FUNCTION_BLOCK FB62
TITLE =Set Position Must
//*****************************************************************************
//* maxon motor ag
//* R&D
//* all rights reserved
//*****************************************************************************
//* Summary:  Write demand value of position
//*
//* Remarks:
//*
//* Created under: STEP7 REV5.2+SP1
//*****************************************************************************
//* History:
//* 18.05.2004 | INA   first release
//*
//*
//*****************************************************************************
//

AUTHOR:INA
FAMILY:PosMode
NAME:SetPosMu
VERSION:00.01


VAR_INPUT

Write : BOOL //A rising edge start the command

  NodeID : BYTE //Adress of the maxon device

  PositionMust : DINT //Position demand value

END_VAR
VAR_OUTPUT
  Done : BOOL //Data valid flag is TRUE if data were available

  Err : BOOL //Error flag is TRUE if an Error has occured, see ErrNo for more details

  ErrNo : DINT //Contains detailed error information

END_VAR
VAR
  xEdgeMerker : BOOL //Edge Merker

  xEdgeFlag : BOOL //Edge Flag

  xStep : INT
END_VAR

BEGIN

NETWORK
TITLE = Activate the service function
//

// SDO Write "Set Position Must"

       U    #Write
       FP   #xEdgeFlag                   // recognize a positiv edge of the Read signal
       =    #xEdgeMerker                 // and set the xEdgeMerker for one cycle to true

       L    #xStep
       L    0
       ==I
       U    #xEdgeMerker
       SPB  nstp                         // iStep = 1 -> fnc1

       L    #xStep                       // jump list
       SPL  List
       SPA  rdef
       SPA  fnc1
       SPA  fncE
List  :SPA  rdef

rdef  :NOP  0
       R    #Done                        // reset Done
       R    #Err
       L    0
       T    #xStep                       // iStep = 0
       SPA  end

fnc1  :NOP  0
       CALL FC13
         NodeID:=#NodeID
         Index:=DW#16#00002062
         SubIndex:=DW#16#00000000
         ValueIn:=#PositionMust
         RET_VAL:=#Done
         Err:=#Err
         ErrNo:=#ErrNo

fncE  :NOP  0
       L    0
       T    #xStep
       SPA  end

nstp  :NOP  0
       L    #xStep
       INC            1
       T    #xStep

end   :NOP  0
END_FUNCTION_BLOCK
